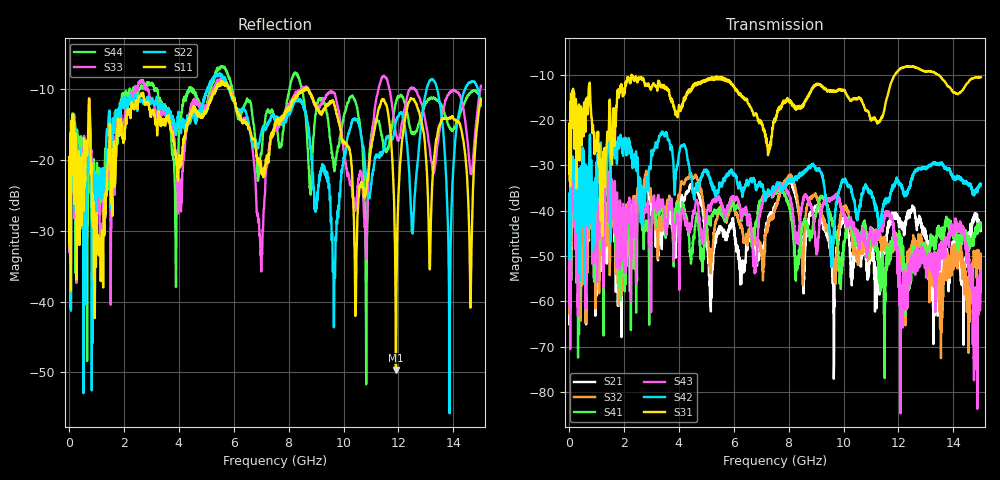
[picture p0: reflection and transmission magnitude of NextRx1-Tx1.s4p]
! FILE: N:\QM 2007\Prüfprotokolle\Highspeed\Konfektionierte Ltg\L45593-D106\D30\8216\0002\Next\NextRx1-Tx1.s4p
# MHz S DB R 50.00
! FREQ  S11  S12  S13  S14
!  S21  S22  S23  S24
!  S31  S32  S33  S34
!  S41  S42  S43  S44
!  DB  ANG  DB  ANG  DB  ANG  DB  ANG
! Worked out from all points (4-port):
!   2999 points, 10 MHz to 15 GHz, reference 50 ohm
!   strongest paths, dB at 10 MHz, 3.755 GHz, 7.505 GHz, 11.26 GHz, 15 GHz:
!     S31: -26.3, -15.4, -20.3, -20.3, -10.5
!     S42: -39.4, -26.1, -35.5, -42.3, -34.1
!     S43: -47.4, -39.4, -35.4, -44.3, -55.6
!     S41: -52.7, -40.0, -36.0, -49.2, -43.2
!     S32: -52.8, -39.5, -39.6, -44.3, -51.3
!     S21: -50.7, -44.0, -38.9, -53.0, -44.3
!   lowest |S11| = -49.6 dB at 11.9 GHz (marker M1), VSWR 1.01, Z = 50.3 - j0.0264 ohm
!   |S11| at or under -10 dB: start of sweep to 5.331 GHz; 5.858 GHz to 8.55 GHz (2.692 GHz wide, 37.4 % of centre); 8.709 GHz to end of sweep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
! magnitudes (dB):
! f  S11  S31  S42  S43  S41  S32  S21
! 10 MHz  -19.6  -26.3  -39.4  -47.4  -52.7  -52.8  -50.7
! 8.665 GHz  -9.8  -15.3  -30.8  -37.1  -43.3  -39.2  -44.1
! 10.45 GHz  -41.4  -15.2  -40.1  -44.5  -46.1  -48.9  -49.4
! 11.44 GHz  -11.4  -18.8  -39.1  -42.5  -52.4  -46.9  -46.6
! 11.9 GHz  -49.6  -9.6  -33.2  -48.3  -46.2  -46.0  -40.9
! 13.86 GHz  -14.0  -12.7  -30.7  -44.7  -42.8  -50.6  -53.4
! 15 GHz  -11.3  -10.5  -34.1  -55.6  -43.2  -51.3  -44.3
